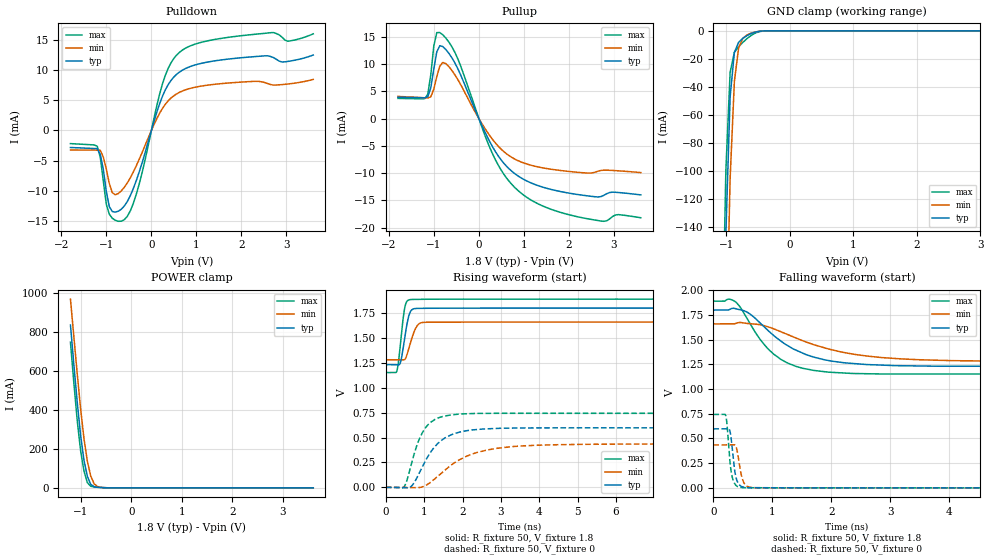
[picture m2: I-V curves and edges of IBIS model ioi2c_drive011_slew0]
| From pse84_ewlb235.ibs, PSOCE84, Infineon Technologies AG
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[Model] ioi2c_drive011_slew0
Model_type I/O
Enable   Active-High
Vinl  =  0.54
Vinh  =  1.26
Vmeas =  0.9
Cref  =  15e-12
| Capacitance   typ   min   max
C_comp   8.55364e-13 8.30808e-13 8.84570e-13
| Variables   typ   min   max
[GND Clamp Reference]   0   0   0
[POWER Clamp Reference]   1.8   1.66   1.89
[Pulldown Reference]   0   0   0
[Pullup Reference]   1.8   1.66   1.89
[Temperature Range]   25   125   -40
[Voltage Range]   1.8   1.66   1.89
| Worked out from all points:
|   slope of the pulldown table from 0 to 0.27 V, typ, clamps not added: 44.3 ohm
|   slope of the pullup table from 0 to 0.27 V, typ, clamps not added: 57.9 ohm
|   GND clamp passes 1 mA (typ) near -0.55 V on its own axis
|   POWER clamp passes 1 mA (typ) near -0.55 V on its own axis
|   falling waveform, R_fixture 50, V_fixture 1.8: 20-80 % time 824ps typ, 1.21ns min, 602ps max; typ from 1.8 V to 1.23 V
|   falling waveform, R_fixture 50, V_fixture 0: 20-80 % time 72.7ps typ, 81.5ps min, 68.1ps max; typ from 0.597 V to 0 V
|   rising waveform, R_fixture 50, V_fixture 1.8: 20-80 % time 146ps typ, 190ps min, 125ps max; typ from 1.23 V to 1.8 V
|   rising waveform, R_fixture 50, V_fixture 0: 20-80 % time 630ps typ, 1.08ns min, 418ps max; typ from 0 V to 0.597 V
[GND Clamp]
| Voltage   I(typ)   I(min)   I(max)
-1.204V   -750.5mA   -844.3mA   -692.2mA
-1.07V    -311.8mA   -416.8mA   -250.3mA
-1.003V   -144.6mA   -236.7mA   -99.35mA
-936.6mV  -47.15mA   -105.3mA   -29.57mA
-869.7mV  -15.32mA   -36.11mA   -15.4mA
-802.8mV  -8.178mA   -12.13mA   -11.32mA
-735.9mV  -5.345mA   -5.294mA   -8.218mA
-669mV    -3.361mA   -2.852mA   -5.471mA
-535.2mV  -838.5uA   -772.4uA   -1.486mA
-401.4mV  -47.36uA   -84.85uA   -76.78uA
3.6V      0A         0A         0A
[POWER Clamp]
| Voltage   I(typ)   I(min)   I(max)
-1.204V   837.3mA    970.7mA    749.2mA
-1.137V   634.9mA    778.2mA    540.5mA
-1.07V    440.1mA    587.4mA    346.5mA
-1.003V   270mA      407mA      190.9mA
-936.6mV  141.8mA    252.7mA    85.92mA
-869.7mV  58.74mA    136.5mA    26.66mA
-802.8mV  18.35mA    60.36mA    8.197mA
-735.9mV  5.885mA    21mA       4.755mA
-669mV    2.866mA    6.628mA    3.138mA
-334.5mV  12.31uA    45.7uA     5.857uA
3.6V      0A         0A         0A
[Pulldown]
| Voltage   I(typ)   I(min)   I(max)
-1.8V     -2.834mA   -3.249mA   -2.184mA
-1.204V   -3.027mA   -3.272mA   -2.632mA
-1.07V    -6.438mA   -4.404mA   -8.33mA
-1.003V   -10.12mA   -6.406mA   -12.25mA
-936.6mV  -12.66mA   -8.803mA   -13.93mA
-802.8mV  -13.58mA   -10.7mA    -14.94mA
-669mV    -13.1mA    -10.04mA   -15.09mA
-401.4mV  -9.649mA   -6.904mA   -12.11mA
248.3mV   5.731mA    3.696mA    7.795mA
558.6mV   9.329mA    6.074mA    12.52mA
1.552V    11.73mA    7.791mA    15.32mA
3.6V      12.55mA    8.493mA    16.08mA
[Pullup]
| Voltage   I(typ)   I(min)   I(max)
-1.8V     3.924mA    4.07mA     3.712mA
-1.137V   4.014mA    3.792mA    4.472mA
-1.07V    5.645mA    3.994mA    8.049mA
-1.003V   9.11mA     5.417mA    13.32mA
-936.6mV  12.27mA    7.722mA    15.78mA
-869.7mV  13.38mA    9.652mA    15.79mA
-735.9mV  12.68mA    10.1mA     14.78mA
-468.3mV  9.148mA    7.158mA    10.95mA
372.4mV   -6.121mA   -4.523mA   -7.639mA
869mV     -10.51mA   -7.709mA   -13.18mA
2.191V    -13.92mA   -9.841mA   -18mA
3.6V      -13.99mA   -9.897mA   -18.18mA
[Ramp]
dV/dt_r   0.358291/0.629742n  0.260726/1.07528n  0.446045/0.418324n
dV/dt_f   0.340724/0.823771n  0.22712/1.20534n  0.442328/0.601922n
R_load = 50
[Falling Waveform]
R_fixture = 50
V_fixture = 1.8
V_fixture_min = 1.66
V_fixture_max = 1.89
| Time   V(typ)   V(min)   V(max)
0s        1.8V       1.66V      1.89V
367.1ps   1.816V     1.662V     1.887V
594.1ps   1.771V     1.663V     1.69V
941ps     1.585V     1.627V     1.399V
1.147ns   1.484V     1.58V      1.3V
1.4ns     1.394V     1.517V     1.23V
2.021ns   1.282V     1.396V     1.169V
3.128ns   1.237V     1.308V     1.152V
6.421ns   1.232V     1.28V      1.153V
800ns     1.232V     1.281V     1.153V
[Falling Waveform]
R_fixture = 50
V_fixture = 0
V_fixture_min = 0
V_fixture_max = 0
| Time   V(typ)   V(min)   V(max)
0s        597.2mV    434.5mV    743.4mV
209.5ps   597mV      434.5mV    731.6mV
232.5ps   596.9mV    434.5mV    634.8mV
284.9ps   565.2mV    434.5mV    243.6mV
322.6ps   376.9mV    434.5mV    102mV
372.1ps   137.1mV    429.9mV    31.9mV
481.6ps   13.02mV    110.9mV    3.074mV
550.9ps   3.383mV    25.81mV    1.753mV
1.118ns   681.7uV    913.1uV    463.7uV
800ns     9.706nV    629.8nV    3.759nV
[Rising Waveform]
R_fixture = 50
V_fixture = 1.8
V_fixture_min = 1.66
V_fixture_max = 1.89
| Time   V(typ)   V(min)   V(max)
0s        1.232V     1.281V     1.153V
287.7ps   1.232V     1.281V     1.168V
331.8ps   1.232V     1.281V     1.268V
388.6ps   1.265V     1.282V     1.471V
477.4ps   1.464V     1.28V      1.77V
551.6ps   1.641V     1.332V     1.869V
661.6ps   1.777V     1.476V     1.886V
859.1ps   1.797V     1.64V      1.888V
1.522ns   1.799V     1.659V     1.89V
800ns     1.8V       1.66V      1.89V
[Rising Waveform]
R_fixture = 50
V_fixture = 0
V_fixture_min = 0
V_fixture_max = 0
| Time   V(typ)   V(min)   V(max)
0s        9.708nV    629.6nV    3.759nV
484.8ps   -3.782mV   -547.5uV   10.36mV
650.1ps   6.094mV    -2.709mV   209.9mV
820.4ps   103.4mV    -2.864mV   434.1mV
1.096ns   309.4mV    32.28mV    627.3mV
1.454ns   473.3mV    144.9mV    708.2mV
1.965ns   558.2mV    285.7mV    737.3mV
2.903ns   591.9mV    392.3mV    743.7mV
5.013ns   597.7mV    431.6mV    743.5mV
50ns      597.2mV    434.5mV    743.4mV
